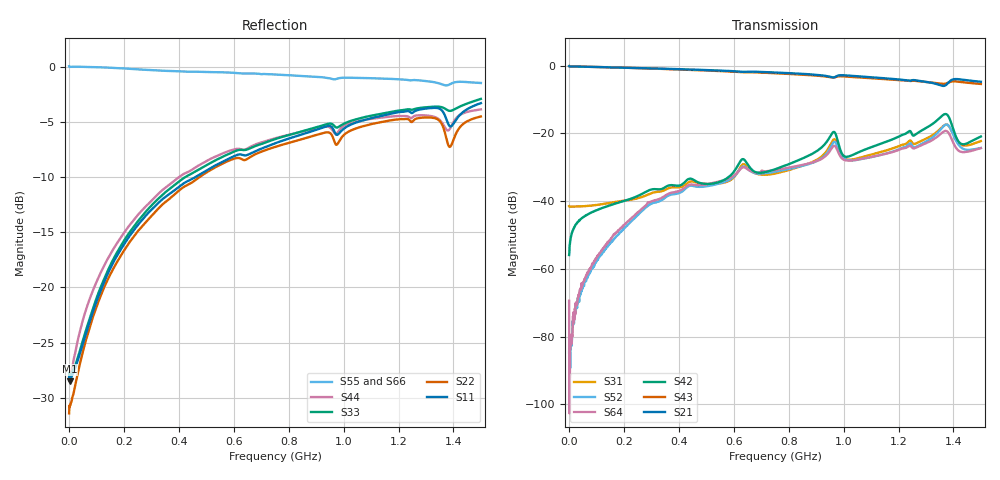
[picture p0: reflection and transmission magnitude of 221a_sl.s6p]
! Generated by Advanced Design System(ADS)'s Touchstone combiner
! Individual SnP file names along with mapping information is saved at the end of this file in XML format
! Created 2019-05-20 11:16:43
# GHz S dB R 50
! 6 Port Network Data
! freq  dBS11  AngS11  dBS12  AngS12  dBS13  AngS13  dBS14  AngS14
!  dBS15  AngS15  dBS16  AngS16
!  dBS21  AngS21  dBS22  AngS22  dBS23  AngS23  dBS24  AngS24
!  dBS25  AngS25  dBS26  AngS26
!  dBS31  AngS31  dBS32  AngS32  dBS33  AngS33  dBS34  AngS34
!  dBS35  AngS35  dBS36  AngS36
!  dBS41  AngS41  dBS42  AngS42  dBS43  AngS43  dBS44  AngS44
!  dBS45  AngS45  dBS46  AngS46
!  dBS51  AngS51  dBS52  AngS52  dBS53  AngS53  dBS54  AngS54
!  dBS55  AngS55  dBS56  AngS56
!  dBS61  AngS61  dBS62  AngS62  dBS63  AngS63  dBS64  AngS64
!  dBS65  AngS65  dBS66  AngS66
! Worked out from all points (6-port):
!   1601 points, 300 kHz to 1.5 GHz, reference 50 ohm
!   strongest paths, dB at 300 kHz, 375.2 MHz, 750.1 MHz, 1.125 GHz, 1.5 GHz:
!     S21: -0.1, -1.0, -2.0, -3.6, -4.7
!     S43: -0.1, -1.1, -2.2, -3.8, -5.4
!     S42: -55.9, -35.3, -30.6, -23.3, -20.9
!     S64: -69.4, -37.5, -30.8, -26.5, -24.3
!     S52: -84.6, -38.0, -31.3, -26.5, -24.3
!     S31: -41.5, -35.9, -31.8, -25.7, -22.2
!   lowest |S11| = -28.5 dB at 2.175 MHz (marker M1), VSWR 1.08, Z = 53.9 - j0.0609 ohm
!   |S11| at or under -10 dB: start of sweep to 459.7 MHz
